(* Logix 5000 AddOnInstructionDefinition export TeNod4TBlocCalibration; software revision 28.00 *)

ADD_ON_INSTRUCTION TeNod4TBlocCalibration   (* revision 1.0, vendor Scaime *)
VAR_IN_OUT
   Datas : TeNod4TDatas; {required}
END_VAR
VAR_INPUT
   NumSegment : INT := 1; {visible}
   ValSegment1 : DINT; {visible}
   ValSegment2 : DINT; {visible}
   ValSegment3 : DINT; {visible}
   Start : BOOL; {visible}
   Zero : BOOL; {visible}
   Segment1 : BOOL; {visible}
   Segment2 : BOOL; {visible}
   Segment3 : BOOL; {visible}
   Save : BOOL; {visible}
   Cancel : BOOL; {visible}
   Theorical : BOOL; {visible}
   ZeroAdjust : BOOL; {visible}
END_VAR
VAR_OUTPUT
   InProgress : BOOL; {visible}
   ZeroDone : BOOL; {visible}
   Seg1Done : BOOL; {visible}
   Seg2Done : BOOL; {visible}
   Seg3Done : BOOL; {visible}
   Complete : BOOL; {visible}
   Error : BOOL; {visible}
END_VAR
VAR
   IntStart1 : BOOL; {access None}
   IntStart2 : BOOL; {access None}
   IntZero : BOOL; {access None}
   IntSeg1 : BOOL; {access None}
   IntSeg2 : BOOL; {access None}
   IntSeg3 : BOOL; {access None}
   IntSave1 : BOOL; {access None}
   IntSave2 : BOOL; {access None}
   IntCancel : BOOL; {access None}
   IntTheo : BOOL; {access None}
   IntZeroA : BOOL; {access None}
   IntSeg1B : BOOL; {access None}
   IntSeg2B : BOOL; {access None}
   IntSeg3B : BOOL; {access None}
END_VAR

ROUTINE Logic   (* ladder *)
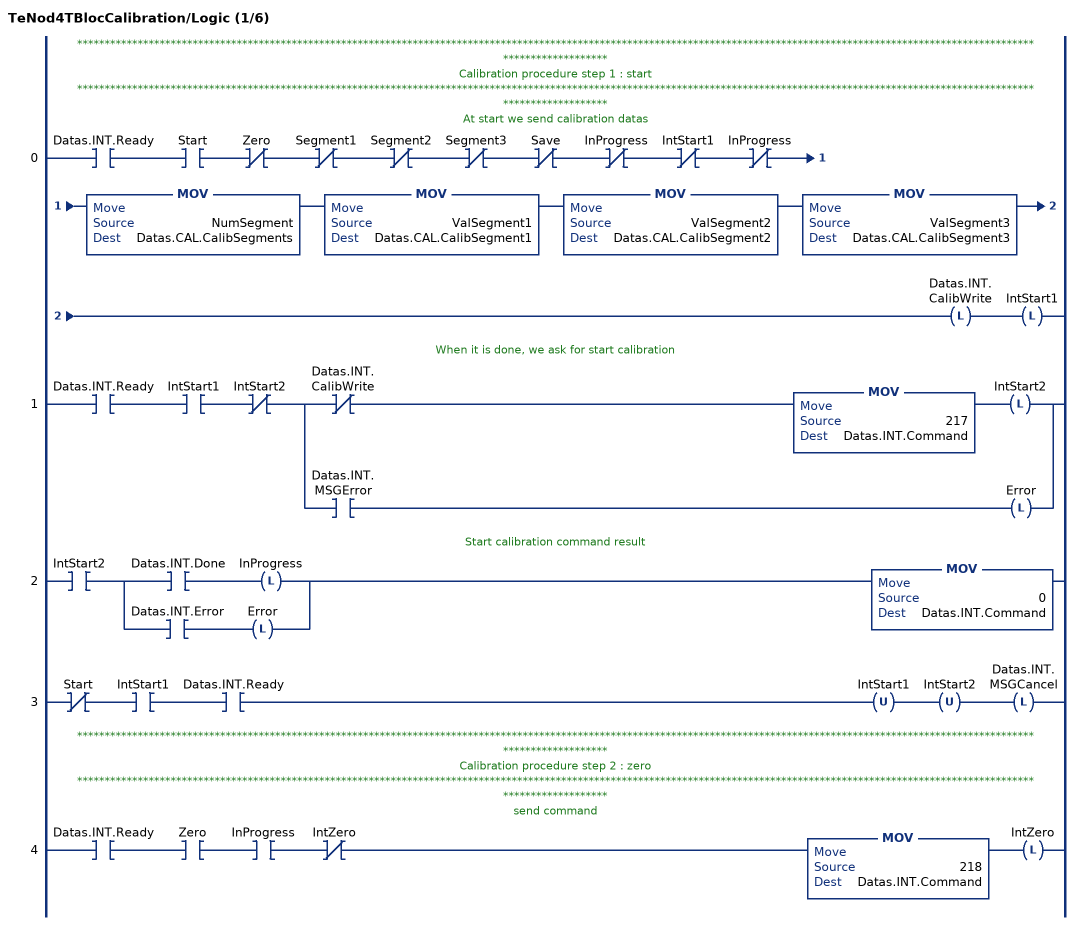
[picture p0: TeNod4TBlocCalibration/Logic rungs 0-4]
   // *************************************************************************************************************************************************************************************************
   // Calibration procedure step 1 : start
   // *************************************************************************************************************************************************************************************************
   // At start we send calibration datas
   0: XIC(Datas.INT.Ready)XIC(Start)XIO(Zero)XIO(Segment1)XIO(Segment2)XIO(Segment3)XIO(Save)XIO(InProgress)XIO(IntStart1)XIO(InProgress)MOV(NumSegment,Datas.CAL.CalibSegments)MOV(ValSegment1,Datas.CAL.CalibSegment1)MOV(ValSegment2,Datas.CAL.CalibSegment2)MOV(ValSegment3,Datas.CAL.CalibSegment3)OTL(Datas.INT.CalibWrite)OTL(IntStart1);
   // When it is done, we ask for start calibration
   1: XIC(Datas.INT.Ready)XIC(IntStart1)XIO(IntStart2)[XIO(Datas.INT.CalibWrite) MOV(217,Datas.INT.Command) OTL(IntStart2) ,XIC(Datas.INT.MSGError) OTL(Error) ];
   // Start calibration command result
   2: XIC(IntStart2)[XIC(Datas.INT.Done) OTL(InProgress) ,XIC(Datas.INT.Error) OTL(Error) ]MOV(0,Datas.INT.Command);
   3: XIO(Start)XIC(IntStart1)XIC(Datas.INT.Ready)OTU(IntStart1)OTU(IntStart2)OTL(Datas.INT.MSGCancel);
   // *************************************************************************************************************************************************************************************************
   // Calibration procedure step 2 : zero
   // *************************************************************************************************************************************************************************************************
   // send command
   4: XIC(Datas.INT.Ready)XIC(Zero)XIC(InProgress)XIO(IntZero)MOV(218,Datas.INT.Command)OTL(IntZero);
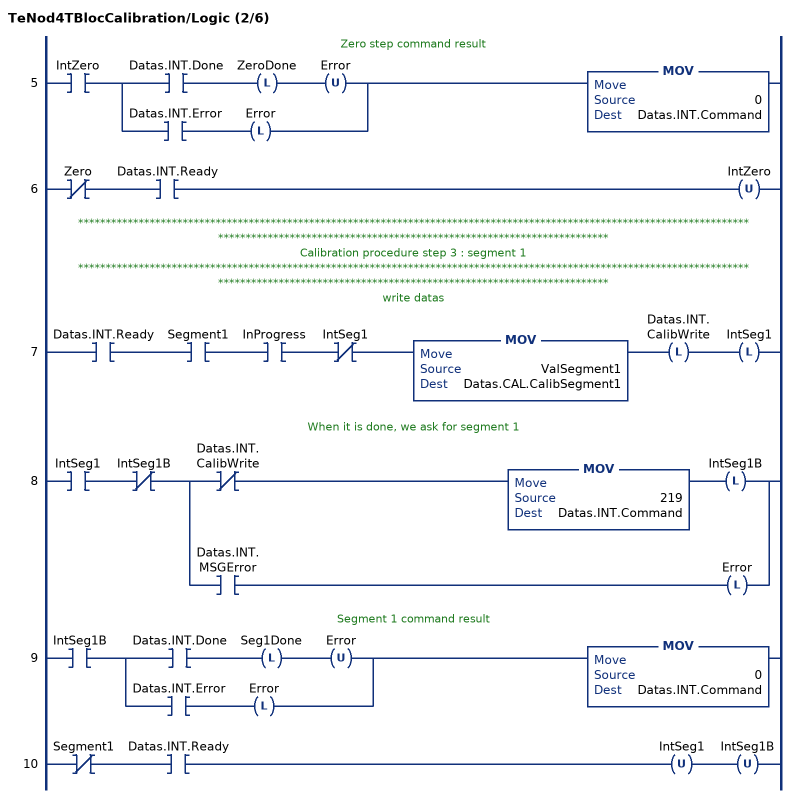
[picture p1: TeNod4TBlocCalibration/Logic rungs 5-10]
   // Zero step command result
   5: XIC(IntZero)[XIC(Datas.INT.Done) OTL(ZeroDone) OTU(Error) ,XIC(Datas.INT.Error) OTL(Error) ]MOV(0,Datas.INT.Command);
   6: XIO(Zero)XIC(Datas.INT.Ready)OTU(IntZero);
   // *************************************************************************************************************************************************************************************************
   // Calibration procedure step 3 : segment 1
   // *************************************************************************************************************************************************************************************************
   // write datas
   7: XIC(Datas.INT.Ready)XIC(Segment1)XIC(InProgress)XIO(IntSeg1)MOV(ValSegment1,Datas.CAL.CalibSegment1)OTL(Datas.INT.CalibWrite)OTL(IntSeg1);
   // When it is done, we ask for segment 1
   8: XIC(IntSeg1)XIO(IntSeg1B)[XIO(Datas.INT.CalibWrite) MOV(219,Datas.INT.Command) OTL(IntSeg1B) ,XIC(Datas.INT.MSGError) OTL(Error) ];
   // Segment 1 command result
   9: XIC(IntSeg1B)[XIC(Datas.INT.Done) OTL(Seg1Done) OTU(Error) ,XIC(Datas.INT.Error) OTL(Error) ]MOV(0,Datas.INT.Command);
   10: XIO(Segment1)XIC(Datas.INT.Ready)OTU(IntSeg1)OTU(IntSeg1B);
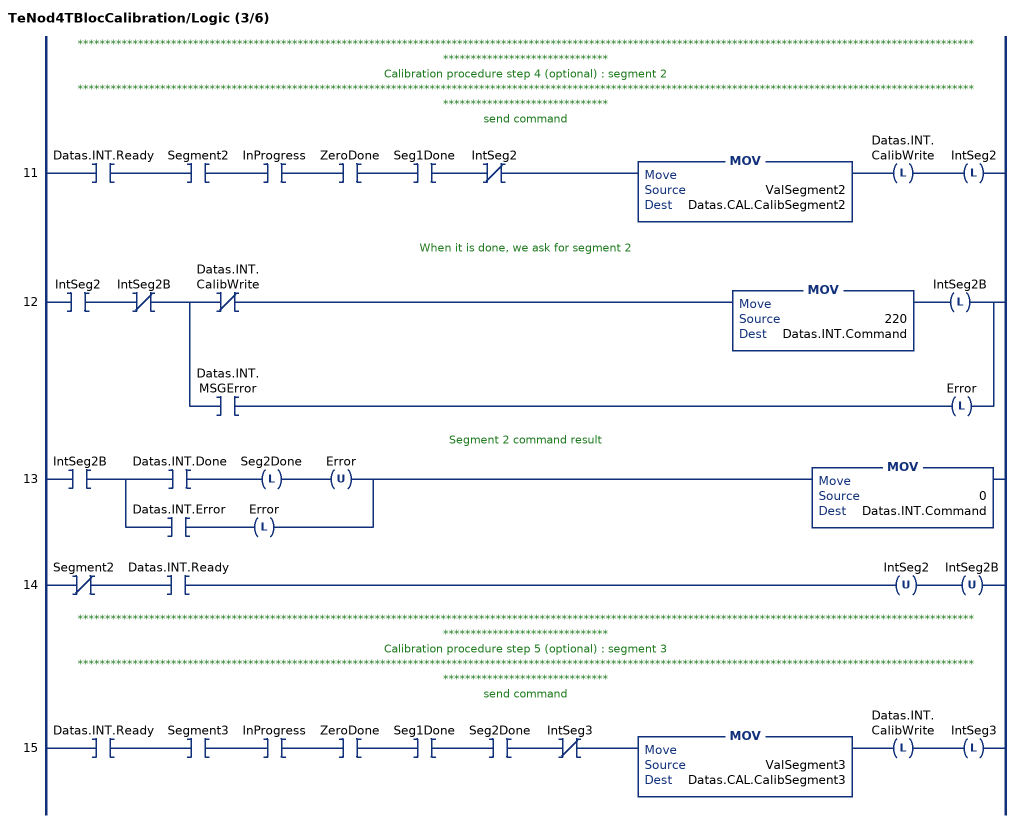
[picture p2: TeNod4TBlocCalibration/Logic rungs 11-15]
   // *************************************************************************************************************************************************************************************************
   // Calibration procedure step 4 (optional) : segment 2
   // *************************************************************************************************************************************************************************************************
   // send command
   11: XIC(Datas.INT.Ready)XIC(Segment2)XIC(InProgress)XIC(ZeroDone)XIC(Seg1Done)XIO(IntSeg2)MOV(ValSegment2,Datas.CAL.CalibSegment2)OTL(Datas.INT.CalibWrite)OTL(IntSeg2);
   // When it is done, we ask for segment 2
   12: XIC(IntSeg2)XIO(IntSeg2B)[XIO(Datas.INT.CalibWrite) MOV(220,Datas.INT.Command) OTL(IntSeg2B) ,XIC(Datas.INT.MSGError) OTL(Error) ];
   // Segment 2 command result
   13: XIC(IntSeg2B)[XIC(Datas.INT.Done) OTL(Seg2Done) OTU(Error) ,XIC(Datas.INT.Error) OTL(Error) ]MOV(0,Datas.INT.Command);
   14: XIO(Segment2)XIC(Datas.INT.Ready)OTU(IntSeg2)OTU(IntSeg2B);
   // *************************************************************************************************************************************************************************************************
   // Calibration procedure step 5 (optional) : segment 3
   // *************************************************************************************************************************************************************************************************
   // send command
   15: XIC(Datas.INT.Ready)XIC(Segment3)XIC(InProgress)XIC(ZeroDone)XIC(Seg1Done)XIC(Seg2Done)XIO(IntSeg3)MOV(ValSegment3,Datas.CAL.CalibSegment3)OTL(Datas.INT.CalibWrite)OTL(IntSeg3);
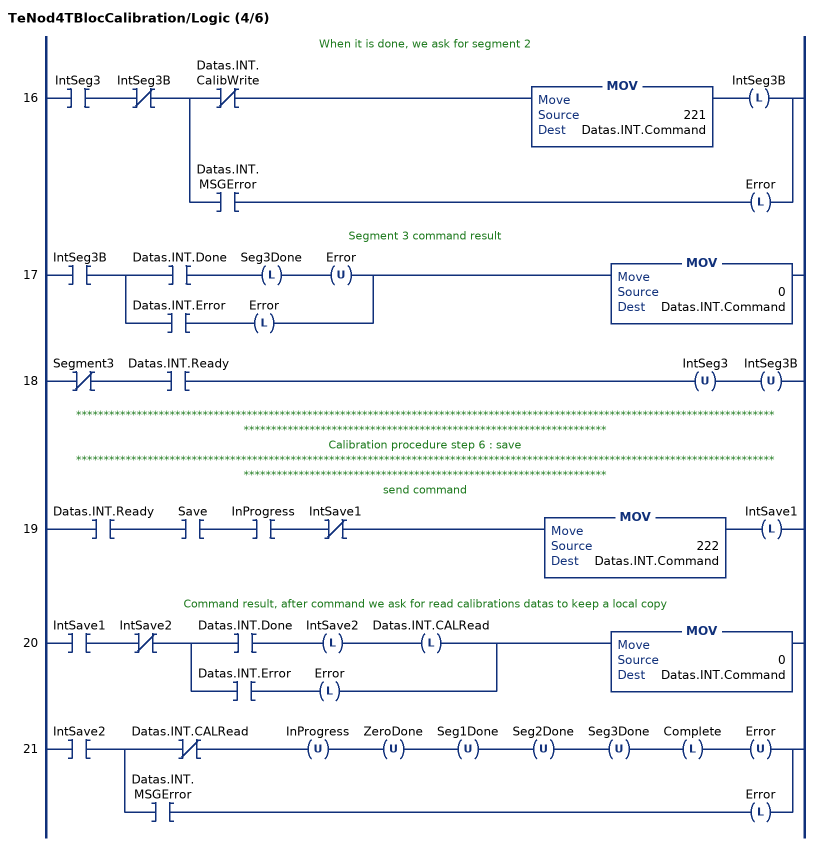
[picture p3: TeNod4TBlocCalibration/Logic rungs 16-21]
   // When it is done, we ask for segment 2
   16: XIC(IntSeg3)XIO(IntSeg3B)[XIO(Datas.INT.CalibWrite) MOV(221,Datas.INT.Command) OTL(IntSeg3B) ,XIC(Datas.INT.MSGError) OTL(Error) ];
   // Segment 3 command result
   17: XIC(IntSeg3B)[XIC(Datas.INT.Done) OTL(Seg3Done) OTU(Error) ,XIC(Datas.INT.Error) OTL(Error) ]MOV(0,Datas.INT.Command);
   18: XIO(Segment3)XIC(Datas.INT.Ready)OTU(IntSeg3)OTU(IntSeg3B);
   // *************************************************************************************************************************************************************************************************
   // Calibration procedure step 6 : save
   // *************************************************************************************************************************************************************************************************
   // send command
   19: XIC(Datas.INT.Ready)XIC(Save)XIC(InProgress)XIO(IntSave1)MOV(222,Datas.INT.Command)OTL(IntSave1);
   // Command result, after command we ask for read calibrations datas to keep a local copy
   20: XIC(IntSave1)XIO(IntSave2)[XIC(Datas.INT.Done) OTL(IntSave2) OTL(Datas.INT.CALRead) ,XIC(Datas.INT.Error) OTL(Error) ]MOV(0,Datas.INT.Command);
   21: XIC(IntSave2)[XIO(Datas.INT.CALRead) OTU(InProgress) OTU(ZeroDone) OTU(Seg1Done) OTU(Seg2Done) OTU(Seg3Done) OTL(Complete) OTU(Error) ,XIC(Datas.INT.MSGError) OTL(Error) ];
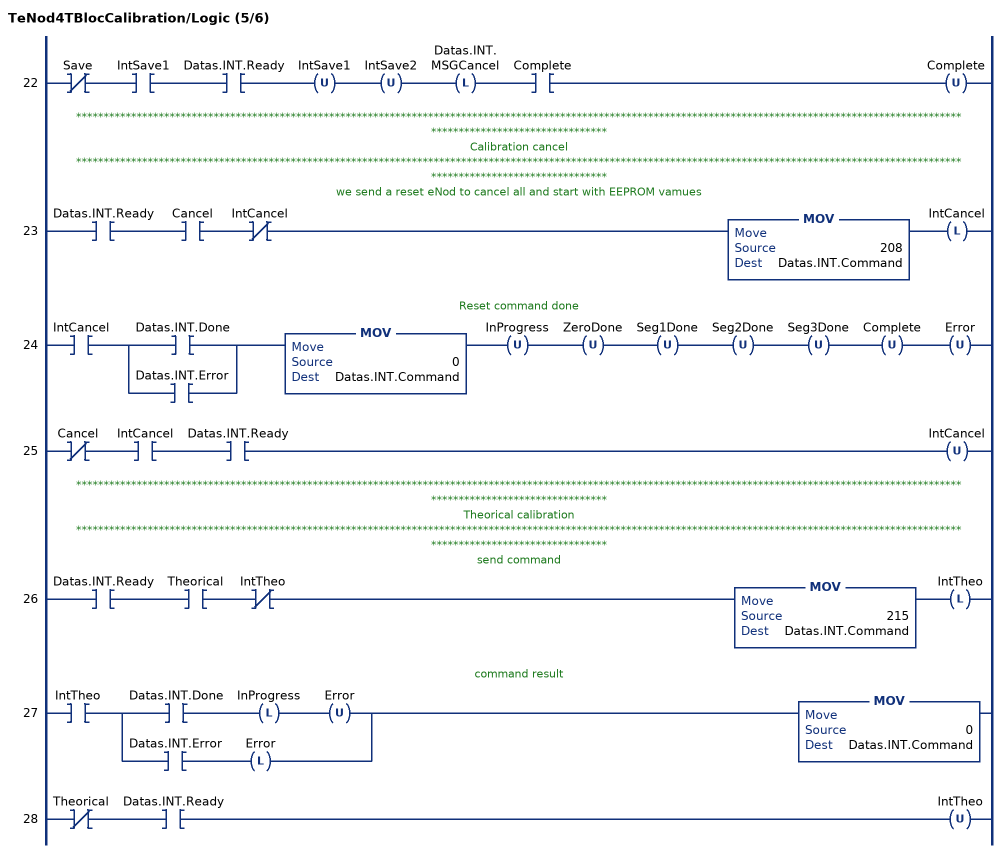
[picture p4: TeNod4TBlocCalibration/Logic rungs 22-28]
   22: XIO(Save)XIC(IntSave1)XIC(Datas.INT.Ready)OTU(IntSave1)OTU(IntSave2)OTL(Datas.INT.MSGCancel)XIC(Complete)OTU(Complete);
   // *************************************************************************************************************************************************************************************************
   // Calibration cancel
   // *************************************************************************************************************************************************************************************************
   // we send a reset eNod to cancel all and start with EEPROM vamues
   23: XIC(Datas.INT.Ready)XIC(Cancel)XIO(IntCancel)MOV(208,Datas.INT.Command)OTL(IntCancel);
   // Reset command done
   24: XIC(IntCancel)[XIC(Datas.INT.Done) ,XIC(Datas.INT.Error) ]MOV(0,Datas.INT.Command)OTU(InProgress)OTU(ZeroDone)OTU(Seg1Done)OTU(Seg2Done)OTU(Seg3Done)OTU(Complete)OTU(Error);
   25: XIO(Cancel)XIC(IntCancel)XIC(Datas.INT.Ready)OTU(IntCancel);
   // *************************************************************************************************************************************************************************************************
   // Theorical calibration
   // *************************************************************************************************************************************************************************************************
   // send command
   26: XIC(Datas.INT.Ready)XIC(Theorical)XIO(IntTheo)MOV(215,Datas.INT.Command)OTL(IntTheo);
   // command result
   27: XIC(IntTheo)[XIC(Datas.INT.Done) OTL(InProgress) OTU(Error) ,XIC(Datas.INT.Error) OTL(Error) ]MOV(0,Datas.INT.Command);
   28: XIO(Theorical)XIC(Datas.INT.Ready)OTU(IntTheo);
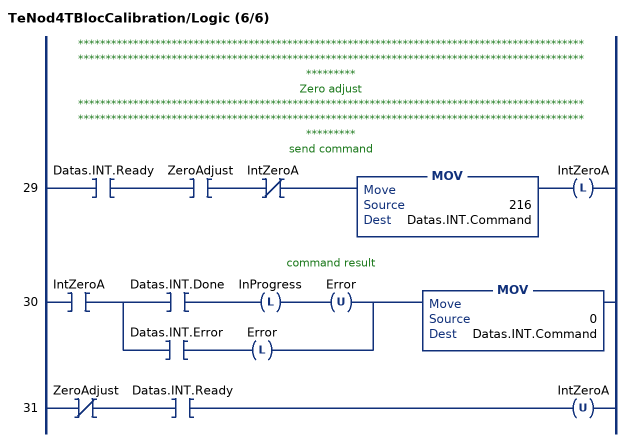
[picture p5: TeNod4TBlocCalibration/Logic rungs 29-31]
   // *************************************************************************************************************************************************************************************************
   // Zero adjust
   // *************************************************************************************************************************************************************************************************
   // send command
   29: XIC(Datas.INT.Ready)XIC(ZeroAdjust)XIO(IntZeroA)MOV(216,Datas.INT.Command)OTL(IntZeroA);
   // command result
   30: XIC(IntZeroA)[XIC(Datas.INT.Done) OTL(InProgress) OTU(Error) ,XIC(Datas.INT.Error) OTL(Error) ]MOV(0,Datas.INT.Command);
   31: XIO(ZeroAdjust)XIC(Datas.INT.Ready)OTU(IntZeroA);
END_ROUTINE
END_ADD_ON_INSTRUCTION
